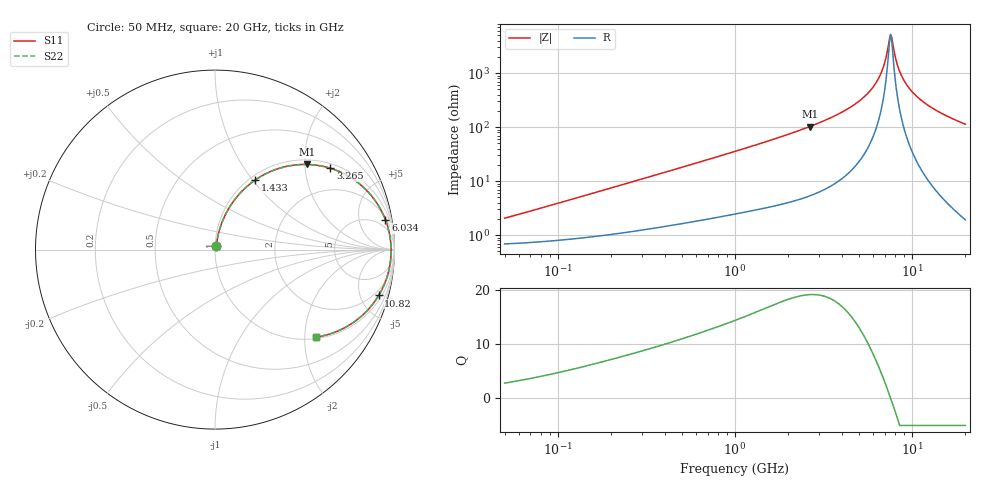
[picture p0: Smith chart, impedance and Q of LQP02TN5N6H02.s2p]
!Murata Part Number: LQP02TN5N6H02
!These Parameters are Measured in Series Mode Connection
!  o--[Z]--o
!Port1  Port2
!  o-------o
!Freq. Start=50[MHz] Stop=20[GHz], 401[Steps]
# Hz S RI R 50
!Freq.(Hz) S11(Real) S11(Imag) S21(Real) S21(Imag) S12(Real) S12(Imag) S22(Real) S22(Imag)
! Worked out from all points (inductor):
!   401 points, 50 MHz to 20 GHz, reference 50 ohm
!   read as one part in series: L = 6.15 nH near 53.89 MHz
!   highest Q = 19.2 at 2.647 GHz (marker M1), where L = 6.18 nH
!   self-resonance near 7.554 GHz
!   S11 on the Smith chart (normalised r, x): 50 MHz: 1.01, +0.04; 1.433 GHz: 1.06, +1.03; 3.265 GHz: 1.15, +2.72; 6.034 GHz: 2, +11; 10.82 GHz: 1.41, -7.01; 20 GHz: 1.04, -2.27
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5e7  0.00723 0.0192  0.9928 -0.0192  0.9928 -0.0192  0.00723 0.0192
1.364002e8  0.0114 0.0505  0.9886 -0.0505  0.9886 -0.0505  0.0114 0.0505
3.721004e8  0.031 0.1291  0.969 -0.1291  0.969 -0.1291  0.031 0.1291
1e9  0.1287 0.3019  0.8713 -0.3019  0.8713 -0.3019  0.1287 0.3019
1.432596e9  0.2224 0.3866  0.7776 -0.3866  0.7776 -0.3866  0.2224 0.3866
2.647493e9  0.5135 0.4744  0.4865 -0.4744  0.4865 -0.4744  0.5135 0.4744
2.728004e9  0.5316 0.4736  0.4684 -0.4736  0.4684 -0.4736  0.5316 0.4736
3.265178e9  0.6432 0.4532  0.3568 -0.4532  0.3568 -0.4532  0.6432 0.4532
4.748272e9  0.8589 0.3149  0.1411 -0.3149  0.1411 -0.3149  0.8589 0.3149
5.433528e9  0.9164 0.2355  0.0836 -0.2355  0.0836 -0.2355  0.9164 0.2355
6.034176e9  0.9497 0.1657  0.0503 -0.1657  0.0503 -0.1657  0.9497 0.1657
6.406762e9  0.9636 0.1234  0.0364 -0.1234  0.0364 -0.1234  0.9636 0.1234
6.802353e9  0.9736 0.0798  0.0264 -0.0798  0.0264 -0.0798  0.9736 0.0798
7.009217e9  0.977 0.0577  0.023 -0.0577  0.023 -0.0577  0.977 0.0577
7.442007e9  0.9809 0.013  0.0191 -0.013  0.0191 -0.013  0.9809 0.013
7.668323e9  0.9812 -0.00952  0.0188 0.00952  0.0188 0.00952  0.9812 -0.00952
8.264682e9  0.9776 -0.0656  0.0224 0.0656  0.0224 0.0656  0.9776 -0.0656
8.907419e9  0.9674 -0.1209  0.0326 0.1209  0.0326 0.1209  0.9674 -0.1209
9.745021e9  0.9469 -0.1851  0.0531 0.1851  0.0531 0.1851  0.9469 -0.1851
1.082228e10  0.9122 -0.2552  0.0878 0.2552  0.0878 0.2552  0.9122 -0.2552
1.417136e10  0.7791 -0.4001  0.2209 0.4001  0.2209 0.4001  0.7791 -0.4001
2e10  0.561 -0.4878  0.439 0.4878  0.439 0.4878  0.561 -0.4878
